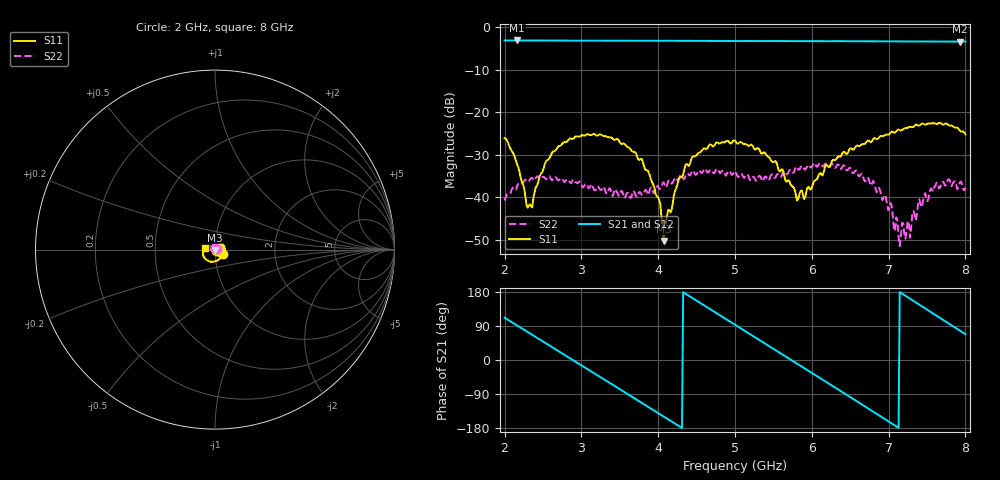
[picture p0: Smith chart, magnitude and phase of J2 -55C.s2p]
!Agilent Technologies,E8364B,MY43040699,A.07.50.67
!Agilent E8364B: A.07.50.67
!Date: Friday, June 06, 2025 09:13:04
!Correction: S11(Full 2 Port(1,2))
!S21(Full 2 Port(1,2))
!S12(Full 2 Port(1,2))
!S22(Full 2 Port(1,2))
!S2P File: Measurements: S11, S21, S12, S22:
# Hz S  dB  R 50
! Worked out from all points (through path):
!   401 points, 2 GHz to 8 GHz, reference 50 ohm
!   highest |S21| = -3.17 dB at 2.165 GHz (marker M1); lowest = -3.5 dB at 7.925 GHz (marker M2)
!   group delay of S21, straight-line fit = 353 ps
!   lowest |S11| = -50.2 dB at 4.07 GHz (marker M3), VSWR 1.01, Z = 49.7 - j0.163 ohm
!   |S11| at or under -10 dB: start of sweep to end of sweep
!   |S22| runs from -51.4 to -31.9 dB; largest |S21 - S12| = 0.0033
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2e9  -26.07 -32.7  -3.18 111.6  -3.19 111.7  -40.71 15.8
2.165e9  -32.38 -42.5  -3.17 90.8  -3.19 90.9  -37.14 -24.0
2.33e9  -41.59 14.0  -3.19 70.0  -3.19 70.1  -35.73 -54.8
2.615e9  -29.59 61.1  -3.20 34.2  -3.20 34.2  -36.00 -108.3
3.005e9  -25.37 24.3  -3.22 -14.8  -3.23 -14.8  -37.20 -177.3
3.53e9  -27.46 -32.5  -3.24 -80.8  -3.26 -80.7  -38.52 117.0
3.785e9  -30.96 -64.5  -3.25 -113.0  -3.26 -112.9  -39.38 96.0
4.01e9  -40.39 -110.0  -3.24 -141.4  -3.27 -141.3  -37.92 85.2
4.07e9  -50.22 -147.9  -3.25 -149.0  -3.27 -148.8  -36.41 86.7
4.265e9  -35.88 86.2  -3.26 -173.6  -3.28 -173.5  -35.70 73.4
4.46e9  -30.39 51.0  -3.27 161.8  -3.29 161.9  -33.73 49.2
5e9  -26.67 -22.7  -3.30 93.4  -3.31 93.6  -33.80 -27.0
5.255e9  -28.73 -57.0  -3.31 61.0  -3.31 61.3  -35.41 -84.0
5.555e9  -32.76 -110.2  -3.31 22.9  -3.32 23.1  -34.45 -145.0
5.81e9  -40.73 178.7  -3.32 -9.6  -3.32 -9.4  -33.03 163.3
6.005e9  -37.37 94.8  -3.33 -34.5  -3.33 -34.3  -32.70 141.2
6.5e9  -28.46 3.6  -3.34 -97.9  -3.36 -97.7  -33.06 86.1
7.01e9  -25.17 -60.4  -3.38 -163.5  -3.38 -163.4  -42.56 72.1
7.16e9  -24.30 -81.2  -3.40 177.1  -3.39 177.3  -49.13 96.9
7.61e9  -22.67 -137.9  -3.43 118.9  -3.41 119.0  -37.19 141.6
7.925e9  -24.27 -178.7  -3.45 77.9  -3.42 78.1  -36.61 97.5
8e9  -25.22 170.3  -3.44 68.1  -3.43 68.2  -37.75 87.9
